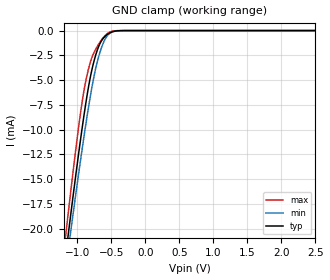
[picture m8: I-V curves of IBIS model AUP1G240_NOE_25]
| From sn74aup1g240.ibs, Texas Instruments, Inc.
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[Model]   AUP1G240_NOE_25
Model_type  Input
Vinl=0.7
Vinh=1.6
| variable   typ   min   max
C_comp   1.63pF   1.37pF   1.94pF
[Temperature Range]   40   100   -40
| Ambient temperature   25   85   -40
[Voltage range]   2.5   2.3   2.7
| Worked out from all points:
|   GND clamp passes 1 mA (typ) near -0.64 V on its own axis
[GND Clamp]
| AUP1G240_NOE_25
|   Voltage   I(typ)   I(min)   I(max)
-3.6V     -171.6mA   -163.5mA   -181.1mA
-1.165V   -22.5mA    -23.95mA   -20.48mA
-1.115V   -19.72mA   -21.35mA   -17.49mA
-1.09V    -18.36mA   -20.06mA   -16.01mA
-945mV    -10.75mA   -12.84mA   -8.061mA
-890mV    -8.117mA   -10.26mA   -5.698mA
-835mV    -5.768mA   -7.825mA   -3.925mA
-760mV    -3.287mA   -4.89mA    -2.329mA
-675mV    -1.463mA   -2.419mA   -1.277mA
-595mV    -617.7uA   -945.8uA   -546.7uA
-520mV    -233.1uA   -272.6uA   -149.9uA
2.5V      104.3pA    491.9pA    26.71pA
